(* 	
	Program Name: 	ACS_MOVE_NO_ACTION
	Purpose:		Prevents motion from occuring
	When Executed:	Primes Output Registers for no action
*)
PROGRAM ACS_MOVE_NO_ACTION
VAR_IN_OUT
	Axis:ACS_DRIVE_TYPE;
END_VAR

VAR_INPUT

END_VAR

VAR
	_moveType:UDINT := ACS_MOTION_TYPES.NO_ACTION;
	// Target Index
	_moveSelect:USINT := 0;
END_VAR

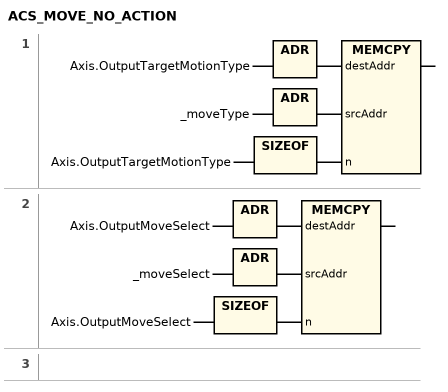
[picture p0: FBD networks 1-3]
// NETWORK 1
MEMCPY(destAddr := ADR(Axis.OutputTargetMotionType), srcAddr := ADR(_moveType), n := SIZEOF(Axis.OutputTargetMotionType));

// NETWORK 2
MEMCPY(destAddr := ADR(Axis.OutputMoveSelect), srcAddr := ADR(_moveSelect), n := SIZEOF(Axis.OutputMoveSelect));

// NETWORK 3

END_PROGRAM
